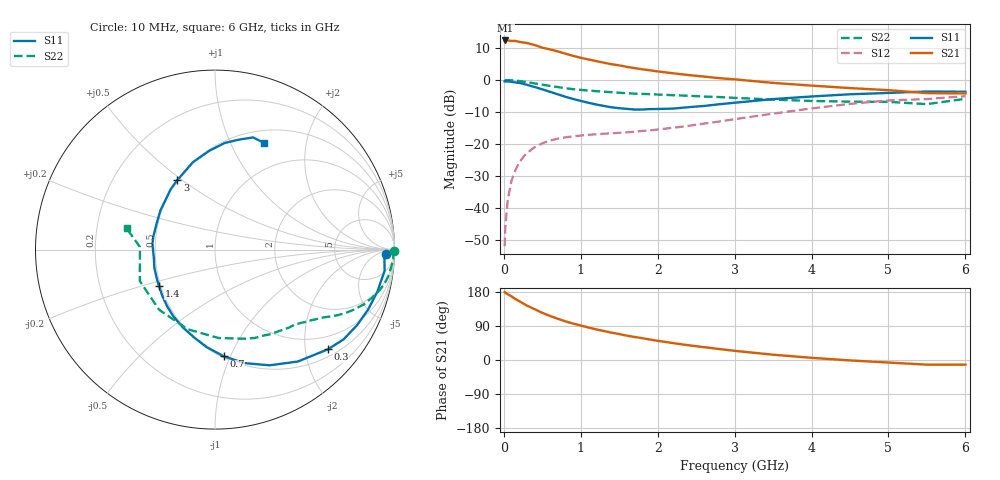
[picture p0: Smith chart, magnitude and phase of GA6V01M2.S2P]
! Infineon Technologies  Discrete & RF Semiconductors
! BF775
! Si NPN RF Bipolar Junction Transistor in SOT23
! VCE = 6 V  IC = 1.2 mA
! Common Emitter S-Parameters:  May  1996
# GHz  S  MA  R  50
!  f  S11  S21  S12  S22
! GHz  MAG  ANG  MAG  ANG  MAG  ANG  MAG  ANG
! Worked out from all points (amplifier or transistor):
!   36 points, 10 MHz to 6 GHz, reference 50 ohm
!   highest |S21| = 12.4 dB at 20 MHz (marker M1)
!   |S21| within 3 dB of that: start of sweep to 632 MHz
!   unconditionally stable (mu >= 1): 1.397 GHz to 3.584 GHz; 5.359 GHz to 5.882 GHz
!   at 250 MHz: K = 0.22, MSG = 18.0 dB, |S12| = -24.2 dB
!   at 1.4 GHz: K = 1.00, MAG = 10.6 dB, |S12| = -16.7 dB
!   at 6 GHz: K = 0.99, MSG = 0.4 dB, |S12| = -5.1 dB
!   S11 on the Smith chart (normalised r, x): 10 MHz: 32, -16; 300 MHz: 0.66, -2.49; 700 MHz: 0.51, -0.95; 1.4 GHz: 0.49, -0.23; 3 GHz: 0.50, +0.48; 6 GHz: 0.64, +1.34
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0.01  0.9514 -1.4  4.082 179.1  0.0025 89.7  0.9999 -0.5
0.02  0.9451 -3.0  4.154 177.4  0.005 87.8  0.9912 -1.1
0.05  0.9525 -7.1  4.15 173.8  0.0131 86.3  0.9955 -2.9
0.1  0.9344 -14.5  4.077 167.9  0.0266 81.7  0.9862 -5.8
0.15  0.9162 -21.4  4.089 160.8  0.0388 76.7  0.9769 -8.8
0.3  0.839 -41.5  3.793 143.5  0.0717 65.7  0.9249 -16.1
0.4  0.7758 -53.5  3.516 134.1  0.0886 59.3  0.8833 -20.2
0.5  0.713 -64.7  3.204 124.4  0.102 54.1  0.8423 -23.4
0.6  0.6532 -75.5  3.008 116.3  0.1128 49.7  0.8076 -26.0
0.7  0.5965 -85.3  2.803 108.9  0.1204 46.5  0.774 -28.2
0.8  0.5455 -94.8  2.583 102.1  0.1264 43.7  0.7425 -30.1
0.9  0.5046 -103.0  2.383 96.1  0.1312 41.9  0.7173 -31.7
1.1  0.4387 -121.8  2.095 85.8  0.1386 39.5  0.6821 -34.7
1.4  0.3729 -146.8  1.765 72.1  0.1461 38.5  0.6431 -38.9
1.7  0.3444 -171.0  1.533 60.8  0.1547 40.7  0.6101 -43.2
2.2  0.3563 155.8  1.271 44.6  0.1785 44.6  0.577 -51.9
3  0.4399 118.6  1.022 24.2  0.2434 47.6  0.5248 -71.2
3.5  0.5021 104.2  0.9 14.0  0.2972 45.4  0.4928 -87.8
4.5  0.5969 84.7  0.746 -1.1  0.4222 34.4  0.4573 -132.9
5  0.6266 77.8  0.692 -6.7  0.4774 26.3  0.454 -157.2
5.5  0.6599 71.3  0.623 -12.3  0.5024 17.0  0.4185 178.0
6  0.6543 65.6  0.615 -12.3  0.5567 12.1  0.5064 166.5
